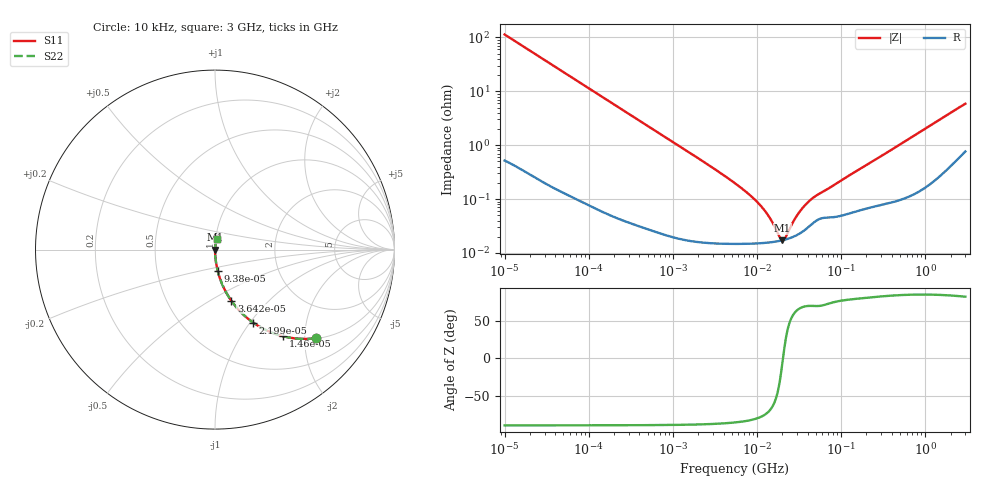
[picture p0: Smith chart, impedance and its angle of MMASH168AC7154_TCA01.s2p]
! MMASH168AC7154_TCA01  S-PARAMETER MODEL  ( Standard Model )
! Model Generated by TAIYO YUDEN Corporation (http://www.ty-top.com)
! Version 1.0
! TAIYO YUDEN Control No. 220601
! Copyright(c) 2019 TAIYO YUDEN CO.,LTD. All Rights Reserved.
! Product Description (link to TY-COMPAS)
! https://ds.yuden.co.jp/TYCOMPAS/or/detail?pn=MMASH168AC7154KTCA01&u=M
! Products Name : Multilayer Ceramic Capacitors
! Characteristics :
!  Capacitance : 0.15 [uF] , Rated Voltage : 100 [V] , TCC : X7S
!  Case Size : 1.6 x 0.8 / 0.063 x 0.031 [mm/inch] , Thickness : 0.8 / 0.031 [mm/inch]
!  (Conditions: Temperature = 25 [degC] , DC Bias Voltage = 0 [V])
! External Node Assignments :
!  1  o---| |---o  2
! GND o---------o GND
! Frequency Range : 10kHz  -  3GHz  [ 401 STEP ]
# MHZ S RI R 50
! Freq[MHz].  S11 Real  S11 Imag  S21 Real  S21 Imag  S12 Real  S12 Imag  S22 Real  S22 Imag
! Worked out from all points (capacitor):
!   401 points, 10 kHz to 3 GHz, reference 50 ohm
!   read as one part in series: C = 140 nF near 10.65 kHz
!   lowest |Z| = 17.3 mohm at 19.95 MHz (marker M1)
!   series resonance near 20.36 MHz, so ESL is about 440 pH
!   S11 on the Smith chart (normalised r, x): 10 kHz: 1.01, -2.27; 14.6 kHz: 1.01, -1.56; 22 kHz: 1.01, -1.03; 36.42 kHz: 1.00, -0.63; 93.8 kHz: 1.00, -0.24; 3 GHz: 1.02, +0.12
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0.01  0.5627 -0.4938  0.4373 0.4938  0.4373 0.4938  0.5627 -0.4938
0.014599  0.3779 -0.4824  0.6221 0.4824  0.6221 0.4824  0.3779 -0.4824
0.021995  0.2123 -0.4065  0.7877 0.4065  0.7877 0.4065  0.2123 -0.4065
0.036425  0.0904 -0.2841  0.9096 0.2841  0.9096 0.2841  0.0904 -0.2841
0.082683  0.0196 -0.1354  0.9804 0.1354  0.9804 0.1354  0.0196 -0.1354
0.093797  0.0154 -0.1199  0.9846 0.1199  0.9846 0.1199  0.0154 -0.1199
0.219733  0.00315 -0.052  0.9968 0.052  0.9968 0.052  0.00315 -0.052
0.683653  0.000517 -0.0168  0.9995 0.0168  0.9995 0.0168  0.000517 -0.0168
2.652321  0.000171 -0.00429  0.9998 0.00429  0.9998 0.00429  0.000171 -0.00429
5.477226  0.000151 -0.00196  0.9998 0.00196  0.9998 0.00196  0.000151 -0.00196
8.516475  0.00015 -0.00112  0.9999 0.00112  0.9999 0.00112  0.00015 -0.00112
11.67315  0.000153 -0.000666  0.9998 0.000666  0.9998 0.000666  0.000153 -0.000666
14.55585  0.000158 -0.000389  0.9998 0.000389  0.9998 0.000389  0.000158 -0.000389
18.73182  0.000168 -9.49e-05  0.9998 9.49e-05  0.9998 9.49e-05  0.000168 -9.49e-05
19.95104  0.000171 -2.31e-05  0.9998 2.31e-05  0.9998 2.31e-05  0.000171 -2.31e-05
21.93027  0.000178 8.46e-05  0.9998 -8.46e-05  0.9998 -8.46e-05  0.000178 8.46e-05
27.34599  0.000201 0.00034  0.9998 -0.00034  0.9998 -0.00034  0.000201 0.00034
32.0153  0.000228 0.000531  0.9998 -0.000531  0.9998 -0.000531  0.000228 0.000531
37.4819  0.000271 0.000729  0.9997 -0.000729  0.9997 -0.000729  0.000271 0.000729
45.28751  0.000347 0.000964  0.9997 -0.000964  0.9997 -0.000964  0.000347 0.000964
374.4521  0.000901 0.00772  0.9991 -0.00772  0.9991 -0.00772  0.000901 0.00772
3000  0.0109 0.0573  0.9891 -0.0573  0.9891 -0.0573  0.0109 0.0573
